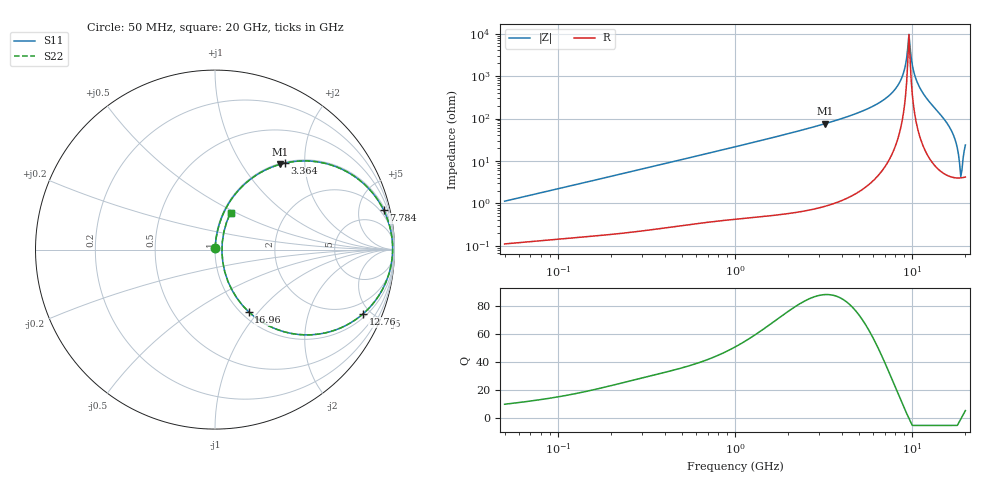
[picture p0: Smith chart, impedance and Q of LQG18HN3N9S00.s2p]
!Murata Part Number: LQG18HN3N9S00
!These Parameters are Measured in Series Mode Connection
!  o--[Z]--o
!Port1  Port2
!  o-------o
!Freq. Start=50[MHz] Stop=20[GHz], 401[Steps]
# Hz S RI R 50
!Freq.(Hz) S11(Real) S11(Imag) S21(Real) S21(Imag) S12(Real) S12(Imag) S22(Real) S22(Imag)
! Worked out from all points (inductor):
!   401 points, 50 MHz to 20 GHz, reference 50 ohm
!   read as one part in series: L = 3.56 nH near 51.52 MHz
!   highest Q = 88 at 3.217 GHz (marker M1), where L = 3.73 nH
!   self-resonance near 9.6 GHz
!   S11 on the Smith chart (normalised r, x): 50 MHz: 1.00, +0.02; 3.364 GHz: 1.02, +1.59; 7.784 GHz: 1.32, +8.44; 12.76 GHz: 1.21, -4.50; 16.96 GHz: 1.08, -0.89; 20 GHz: 1.08, +0.47
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5e7  0.00124 0.0112  0.9988 -0.0112  0.9988 -0.0112  0.00124 0.0112
1.364002e8  0.00251 0.0298  0.9975 -0.0298  0.9975 -0.0298  0.00251 0.0298
3.721004e8  0.00894 0.0797  0.9911 -0.0797  0.9911 -0.0797  0.00894 0.0797
1e9  0.0481 0.2043  0.9519 -0.2043  0.9519 -0.2043  0.0481 0.2043
2.728004e9  0.2809 0.4436  0.7191 -0.4436  0.7191 -0.4436  0.2809 0.4436
3.216634e9  0.364 0.4755  0.636 -0.4755  0.636 -0.4755  0.364 0.4755
3.364474e9  0.3895 0.482  0.6105 -0.482  0.6105 -0.482  0.3895 0.482
5.433528e9  0.7157 0.4437  0.2843 -0.4437  0.2843 -0.4437  0.7157 0.4437
7.442007e9  0.9182 0.259  0.0818 -0.259  0.0818 -0.259  0.9182 0.259
7.784049e9  0.9395 0.2203  0.0605 -0.2203  0.0605 -0.2203  0.9395 0.2203
8.774992e9  0.9799 0.1022  0.0201 -0.1022  0.0201 -0.1022  0.9799 0.1022
9.316812e9  0.9887 0.0355  0.0113 -0.0355  0.0113 -0.0355  0.9887 0.0355
9.600142e9  0.9896 0.00041  0.0104 -0.00041  0.0104 -0.00041  0.9896 0.00041
9.745021e9  0.9891 -0.0175  0.0109 0.0175  0.0109 0.0175  0.9891 -0.0175
1.019291e10  0.9833 -0.0728  0.0167 0.0728  0.0167 0.0728  0.9833 -0.0728
1.066139e10  0.9704 -0.1298  0.0296 0.1298  0.0296 0.1298  0.9704 -0.1298
1.276073e10  0.8241 -0.3586  0.1759 0.3586  0.1759 0.3586  0.8241 -0.3586
1.504638e10  0.5036 -0.4752  0.4964 0.4752  0.4964 0.4752  0.5036 -0.4752
1.696185e10  0.1878 -0.3469  0.8122 0.3469  0.8122 0.3469  0.1878 -0.3469
1.88369e10  0.0387 -0.014  0.9613 0.014  0.9613 0.014  0.0387 -0.014
1.940974e10  0.0494 0.0987  0.9506 -0.0987  0.9506 -0.0987  0.0494 0.0987
2e10  0.0866 0.2055  0.9134 -0.2055  0.9134 -0.2055  0.0866 0.2055
